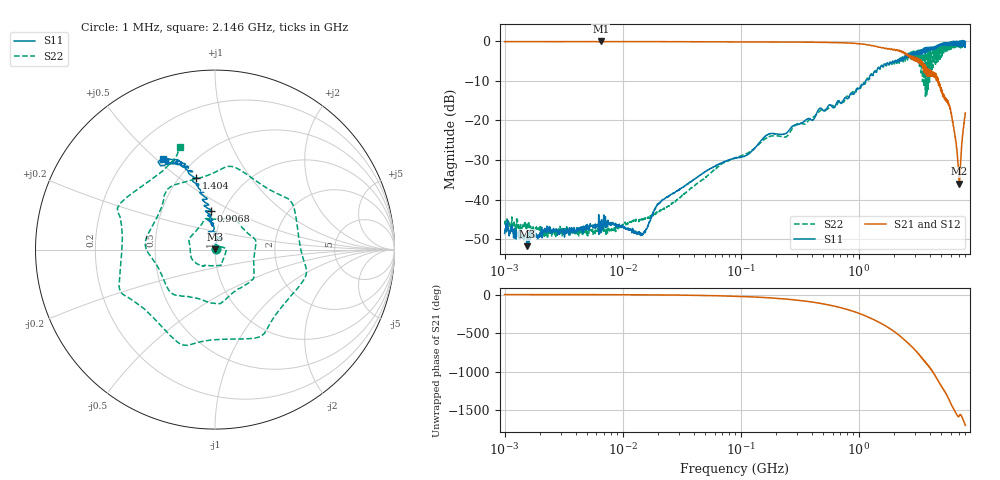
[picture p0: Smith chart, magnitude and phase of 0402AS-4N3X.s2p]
!s-Parameter Generated by FASTRON Sdn. Bhd.
!FASTRON P/N : 0402AS-4N3X
!Keysight Technologies: E5071C_MY46733604_B.14.02
!Date: Mon Dec 01 10:24:01 2025
!Version  :Rev00  Mon Dec 01 10:24:01 2025
!Data & Calibration Information:
!Freq  S11:SOLT2(ON)  S21:SOLT2(ON)  S12:SOLT2(ON)  S22:SOLT2(ON)
!PortZ  Port1:50+j0  Port2:50+j0
!When reading reference impedance value at option line is always used.
! Remarks : This data is being provided solely for informational purposes.
# Hz S dB R 50
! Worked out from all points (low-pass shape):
!   1601 points, 1 MHz to 8 GHz, reference 50 ohm
!   highest |S21| = 0.01 dB at 6.532 MHz (marker M1); lowest = -36.0 dB at 7.113 GHz (marker M2)
!   |S21| within 3 dB of the highest: start of sweep to 2.418 GHz; 2.456 GHz to 2.493 GHz (36.4 MHz wide, 1.47 % of centre)
!   lowest |S11| = -51.8 dB at 1.541 MHz (marker M3), VSWR 1.01, Z = 50.2 + j0.0862 ohm
!   |S11| at or under -10 dB: start of sweep to 1.141 GHz
!   |S22| runs from -49.9 to -0.6 dB; largest |S21 - S12| = 0.017
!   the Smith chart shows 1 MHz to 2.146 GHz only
!   S11 on the Smith chart (normalised r, x): 1 MHz: 1.01, +0.00; 906.8 MHz: 0.88, +0.40; 1.404 GHz: 0.60, +0.58; 2.146 GHz: 0.34, +0.53
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1000000  -48.60 18.3  -0.05 -0.2  -0.04 -0.2  -46.00 18.4
1541011  -51.80 19.5  -0.04 -0.4  -0.03 -0.4  -46.70 -10.0
4479405  -47.00 19.1  -0.05 -1.1  -0.04 -1.2  -48.40 27.8
6531720  -46.70 14.0  0.01 -1.7  -0.04 -1.8  -48.40 23.3
2.00676e7  -41.10 33.5  -0.05 -5.0  -0.05 -4.9  -42.90 56.5
8.994653e7  -29.50 88.5  -0.08 -22.1  -0.08 -22.1  -29.50 24.2
4.006501e8  -19.90 105.0  -0.19 -97.1  -0.19 -97.1  -19.40 -124.0
9.068124e8  -13.30 95.5  -0.47 140.0  -0.47 140.0  -12.80 7.2
1.403687e9  -7.70 105.0  -1.23 20.3  -1.22 20.2  -7.71 113.0
1.7949e9  -5.77 112.0  -1.80 -71.5  -1.80 -71.6  -5.84 -77.6
2.146431e9  -4.67 120.0  -2.42 -156.0  -2.42 -156.0  -4.39 109.0
2.354847e9  -4.40 123.0  -2.76 155.0  -2.74 155.0  -4.01 7.9
2.545586e9  -3.72 125.0  -3.43 109.0  -3.40 109.0  -3.26 -88.0
2.736325e9  -3.15 128.0  -4.18 64.1  -4.15 64.0  -2.72 177.0
2.971081e9  -3.36 137.0  -3.92 8.2  -3.89 8.0  -4.55 61.1
3.26428e9  -3.26 143.0  -4.49 -65.2  -4.46 -65.6  -6.29 -83.8
3.689925e9  -1.56 148.0  -8.23 -158.0  -8.27 -159.0  -7.42 36.1
4.034495e9  -2.00 157.0  -7.65 119.0  -7.71 119.0  -2.41 -83.9
5.136407e9  -0.62 176.0  -13.90 -131.0  -13.90 -132.0  -3.12 96.1
5.500301e9  -0.99 -165.0  -14.70 150.0  -14.80 149.0  -0.91 -78.0
7.113238e9  0.07 -113.0  -36.00 -129.0  -35.90 -130.0  -1.57 -130.0
8e9  -0.01 -91.9  -18.10 106.0  -18.20 105.0  -1.34 149.0
